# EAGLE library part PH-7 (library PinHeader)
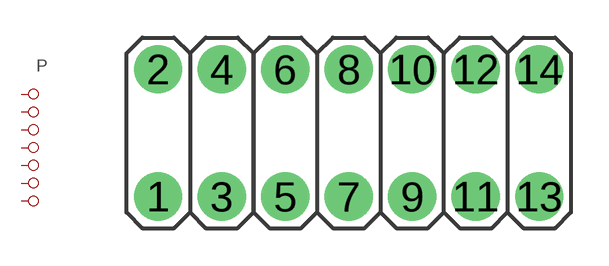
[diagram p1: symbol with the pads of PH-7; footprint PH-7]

Designator prefix P

## PH-7  [PH-7]
1  1  pas
2  1  pas
3  2  pas
4  2  pas
5  3  pas
6  3  pas
7  4  pas
8  4  pas
9  5  pas
10  5  pas
11  6  pas
12  6  pas
13  7  pas
14  7  pas

## Footprint PH-7 (pad centres in mm)
drill 1 pad 1.93: 1 -7.62,-2.54; 2 -7.62,2.54; 3 -5.08,-2.54; 4 -5.08,2.54; 5 -2.54,-2.54; 6 -2.54,2.54; 7 0,-2.54; 8 0,2.54; 9 2.54,-2.54; 10 2.54,2.54; 11 5.08,-2.54; 12 5.08,2.54; 13 7.62,-2.54; 14 7.62,2.54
